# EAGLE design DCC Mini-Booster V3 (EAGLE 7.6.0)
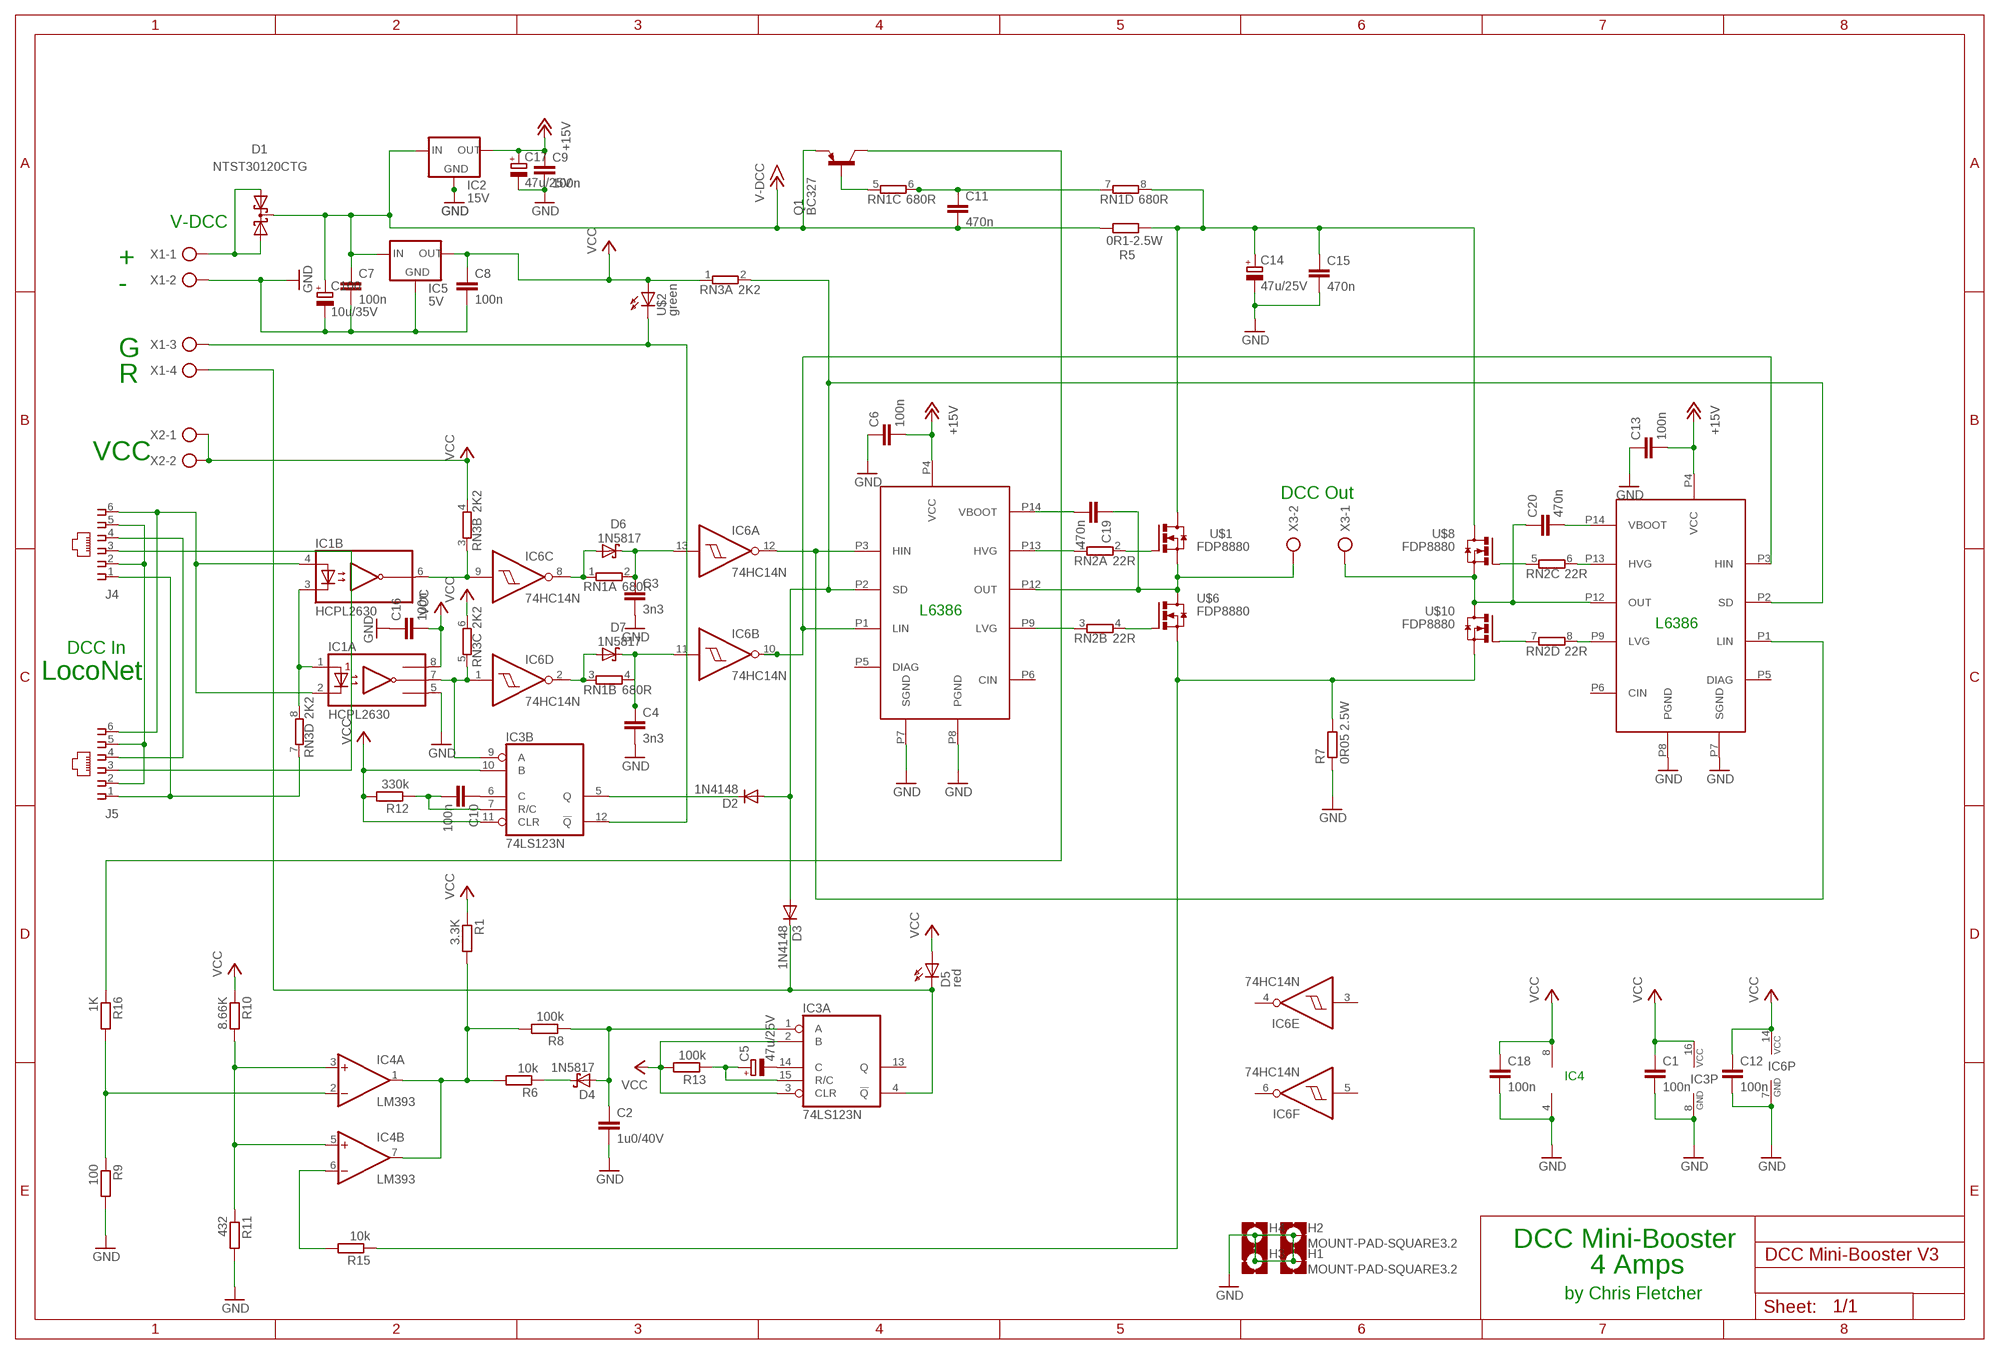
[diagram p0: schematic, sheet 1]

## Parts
C1  100n  C-EU050-025X075  [C050-025X075]
C2  1u0/40V  C5/5.5  [C5B5.5]
C3  3n3  C-EU050-025X075  [C050-025X075]
C4  3n3  C-EU050-025X075  [C050-025X075]
C5  47u/25V  CPOL-EUE2.5-6  [E2,5-6]
C6  100n  C-EU050-025X075  [C050-025X075]
C7  100n  C-EU050-025X075  [C050-025X075]
C8  100n  C-EU050-025X075  [C050-025X075]
C9  100n  C-EU050-025X075  [C050-025X075]
C10  100n  C-EU050-025X075  [C050-025X075]
C11  470n  C-EU050-025X075  [C050-025X075]
C12  100n  C-EU050-025X075  [C050-025X075]
C13  100n  C-EU050-025X075  [C050-025X075]
C14  47u/25V  CPOL-EUE2.5-6  [E2,5-6]
C15  470n  C-EU050-025X075  [C050-025X075]
C16  100n  C-EU050-025X075  [C050-025X075]
C17  47u/25V  CPOL-EUE2.5-6  [E2,5-6]
C18  100n  C-EU050-025X075  [C050-025X075]
C19  470n  C-EU050-025X075  [C050-025X075]
C20  470n  C-EU050-025X075  [C050-025X075]
C100  10u/35V  CPOL-EUE5-4  [E5-4]
D1  NTST30120CTG  DIODE_2SCHOTTKY-SOT82V  [SOT82S]
D2  1N4148  [DO35-10]
D3  1N4148  [DO35-10]
D4  1N5817  1N5817-B  [DO41-7.6]
D5  red  LED3MM  [LED3MM]
D6  1N5817  1N5817-B  [DO41-7.6]
D7  1N5817  1N5817-B  [DO41-7.6]
H1  MOUNT-PAD-SQUARE3.2  [3,2-PAD-SQUARE]
H2  MOUNT-PAD-SQUARE3.2  [3,2-PAD-SQUARE]
H3  MOUNT-PAD-SQUARE3.2  [3,2-PAD-SQUARE]
H4  MOUNT-PAD-SQUARE3.2  [3,2-PAD-SQUARE]
IC1  HCPL2630  [DIL08]
IC2  15V  78XXS  [78XXS]
IC3  74LS123N  [DIL16]
IC4  LM393  [DIL08N]
IC5  5V  78XXS  [78XXS]
IC6  74HC14N  [DIL14]
J4  520258-3  [520258-3]
J5  520258-3  [520258-3]
Q1  BC327  [TO92-EBC]
R1  3.3K  R-EU_0207/10  [0207/10]
R5  0R1-2.5W  R-EU_0613/5V  [P0613V]
R6  10k  R-EU_0207/10  [0207/10]
R7  0R05 2.5W  R-EU_0613/5V  [P0613V]
R8  100k  R-EU_0207/10  [0207/10]
R9  100  R-EU_0207/10  [0207/10]
R10  8.66K  R-EU_0207/10  [0207/10]
R11  432  R-EU_0207/10  [0207/10]
R12  330k  R-EU_0207/10  [0207/10]
R13  100k  R-EU_0207/10  [0207/10]
R15  10k  R-EU_0207/10  [0207/10]
R16  1K  R-EU_0207/10  [0207/10]
RN1  680R  E4R  [SIL8]
RN2  22R  E4R  [SIL8]
RN3  2K2  E4R  [SIL8]
U$1  FDP8880  IRFZ44Z  [TO220AV]
U$2  green  LED3MM  [LED3MM]
U$6  FDP8880  IRFZ44Z  [TO220AV]
U$7  L6386  [DIL14-1]
U$8  FDP8880  IRFZ44Z  [TO220AV]
U$9  L6386  [DIL14-1]
U$10  FDP8880  IRFZ44Z  [TO220AV]
X1  + - G R  AK500/4  [AK500/4]
X2  AK500/2  [AK500/2]
X3  AK500/2  [AK500/2]

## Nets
+12V [+15V]: C6.2 C9.1 C13.2 C17.+ IC2.OUT U$7.P4(VCC) U$9.P4(VCC) ; supply symbol labelled +15V
+15V [+VDCC]: C7.1 C11.2 C100.+ D1.C IC2.IN IC5.IN Q1.E R5.1 ; supply symbol labelled V-DCC
C10: C10.2 IC3.7(B:R/C) R12.1
GND [GND]: C1.2 C2.2 C3.2 C4.2 C6.1 C7.2 C8.2 C9.2 C12.2 C13.1 C14.- C15.2 C16.1 C17.- C18.2 C100.- H1.B3,2(MOUNT) H2.B3,2(MOUNT) H3.B3,2(MOUNT) H4.B3,2(MOUNT) IC1.5(A:GND) IC2.GND IC3.8(P:GND) IC4.4(P:V-) IC5.GND IC6.7(P:GND) R7.1 R9.2 R11.2 U$7.P7(SGND) U$7.P8(PGND) U$9.P7(SGND) U$9.P8(PGND) X1.2
N$1: IC4.1(A:OUT) IC4.7(B:OUT) R1.2 R6.2 R8.2
N$2: D4.C R6.1
N$3: C2.1 D4.A IC3.1(A:A) R8.1
N$4: C11.1 RN1.6 RN1.7
N$5: C20.2 U$9.P14(VBOOT)
N$6 [signal]: D6.A IC6.8(C:O) RN1.1
N$7: C5.- IC3.14(A:C)
N$8 [signal]: C3.1 D6.C IC6.13(A:I) RN1.2
N$9 [+VDCC]: R7.2 R15.1 U$6.E(S) U$10.E(S)
N$10 [signal]: J4.2 J4.5 J5.2 J5.5
N$11 [signal]: IC1.2(A:C1) IC1.4(B:A2) J4.6 J5.6
N$12: IC1.7(A:VO1) IC3.9(B:A) IC6.1(D:I) RN3.5
N$13 [signal]: J4.3 J5.3
N$14 [signal]: J4.1 J5.1 RN3.7
N$15: IC4.3(A:+IN) IC4.5(B:+IN) R10.2 R11.1
N$16 [signal]: J4.4 J5.4
N$17: IC4.6(B:-IN) R15.2
N$18: IC3.12(B:!Q) U$2.K(C) X1.3
N$19: Q1.C R16.1
N$20 [+VDCC]: C19.1 U$1.E(S) U$6.C(D) U$7.P12(OUT) X3.2
N$21: C4.1 D7.C IC6.11(B:I) RN1.4
N$22: D2.A D3.A RN3.2 U$7.P2(SD) U$9.P2(SD)
N$23 [signal]: IC6.12(A:O) U$7.P3(HIN) U$9.P1(LIN)
N$24: IC4.2(A:-IN) R9.1 R16.2
N$26 [+VDCC]: D1.A1 D1.A2 X1.1
N$28: IC1.1(A:A1) IC1.3(B:C2) RN3.8
N$29 [GND]: C14.+ C15.1 R5.2 RN1.8 U$1.C(D) U$8.C(D)
N$31: Q1.B RN1.5
N$32: RN2.2 U$1.B(G)
N$33: D7.A IC6.2(D:O) RN1.3
N$34 [+VDCC]: C20.1 U$8.E(S) U$9.P12(OUT) U$10.C(D) X3.1
N$35 [signal]: IC1.6(B:VO2) IC6.9(C:I) RN3.3
N$37: RN2.1 U$7.P13(HVG)
N$38: C10.1 IC3.6(B:C)
N$39: D2.C IC3.5(B:Q)
N$40: RN2.4 U$6.B(G)
N$41: RN2.3 U$7.P9(LVG)
N$42: RN2.6 U$9.P13(HVG)
N$43: C5.+ IC3.15(A:R/C) R13.1
N$44: RN2.5 U$8.B(G)
N$45: RN2.8 U$9.P9(LVG)
N$46: RN2.7 U$10.B(G)
N$47: D3.C D5.K(C) IC3.4(A:!Q) X1.4
N$48: IC6.10(B:O) U$7.P1(LIN) U$9.P3(HIN)
N$59: C19.2 U$7.P14(VBOOT)
VCC [VCC]: C1.1 C8.1 C12.1 C16.2 C18.1 D5.A IC1.8(A:VCC) IC3.2(A:B) IC3.3(A:CLR) IC3.10(B:B) IC3.11(B:CLR) IC3.16(P:VCC) IC4.8(P:V+) IC5.OUT IC6.14(P:VCC) R1.1 R10.1 R12.2 R13.2 RN3.1 RN3.4 RN3.6 U$2.A X2.1 X2.2
Unconnected: IC3.13(A:Q) IC6.3(E:I) IC6.4(E:O) IC6.5(F:I) IC6.6(F:O) U$7.P5(DIAG) U$7.P6(CIN) U$9.P5(DIAG) U$9.P6(CIN)

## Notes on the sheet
- V-DCC
- +
- -
- G
- R
- VCC
- DCC Out
- L6386
- L6386
- DCC In
- LocoNet
- IC4
- DCC Mini-Booster
- 4 Amps
- by Chris Fletcher

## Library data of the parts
C1 C3 C4 C6-C13 C15 C16 C18-C20 = rcl:C-EU: CAPACITOR, European symbol
C2 = capacitor-wima:C: CAPACITOR
C5 C14 C17 C100 = rcl:CPOL-EU: POLARIZED CAPACITOR, European symbol
D1 = diode:DIODE_2SCHOTTKY-: Dual SCHOTTKY DIODE common cathode
D2 D3 = diode:1N4148: DIODE
D4 D6 D7 = diode:1N581*: 1.0A SCHOTTKY BARRIER RECTIFIER
D5 U$2 = led:LED: LED
H1-H4 = holes:MOUNT-PAD-SQUARE: MOUNTING PAD, square
IC1 = optocoupler:HCPL2630: HEWLETT PACKARD OPTO COUPLER
IC2 IC5 = v-reg:78XXS: VOLTAGE REGULATOR
IC3 = 74xx-eu:74*123: Retriggerable monostable MULTIVIBRATOR
IC4 = linear:LM393: COMPARATOR
IC6 = 74xx-eu:74*14: Hex schmitt trigger INVERTER
J4 J5 = con-amp:520258-3: AMP connector; MF: TYCO ELECTRONICS; MPN: 5520258-3; OC_FARNELL: 1214651; OC_NEWARK: 42K7227
Q1 = transistor-pnp:BC327*: PNP Transistror
R1 R5-R13 R15 R16 = rcl:R-EU_: RESISTOR, European symbol
RN1-RN3 = resistor-sil:E4R: SIL RESISTOR; OC_FARNELL: unknown; OC_NEWARK: unknown
U$1 U$6 U$8 U$10 = transistor-power:IRFZ44Z: N-Channel MOSFET TO-220 Pack
U$7 U$9 = jfw-pwm1:L6386: High and low side MOSFET Driver
X1 = con-ptr500:AK500/4: CONNECTOR; OC_FARNELL: unknown; OC_NEWARK: unknown
X2 X3 = con-ptr500:AK500/2: CONNECTOR; OC_FARNELL: unknown; OC_NEWARK: unknown

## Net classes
1 signal: width 0.381 mm, drill 0.508 mm, clearance 0.381 mm
2 VCC: width 0.635 mm, drill 0.508 mm, clearance 0.381 mm
3 +15V: width 0.635 mm, drill 0.508 mm, clearance 0.381 mm
4 +VDCC: width 1.803 mm, drill 0.762 mm, clearance 0.381 mm
5 GND: width 0.635 mm, drill 0.508 mm, clearance 0.381 mm

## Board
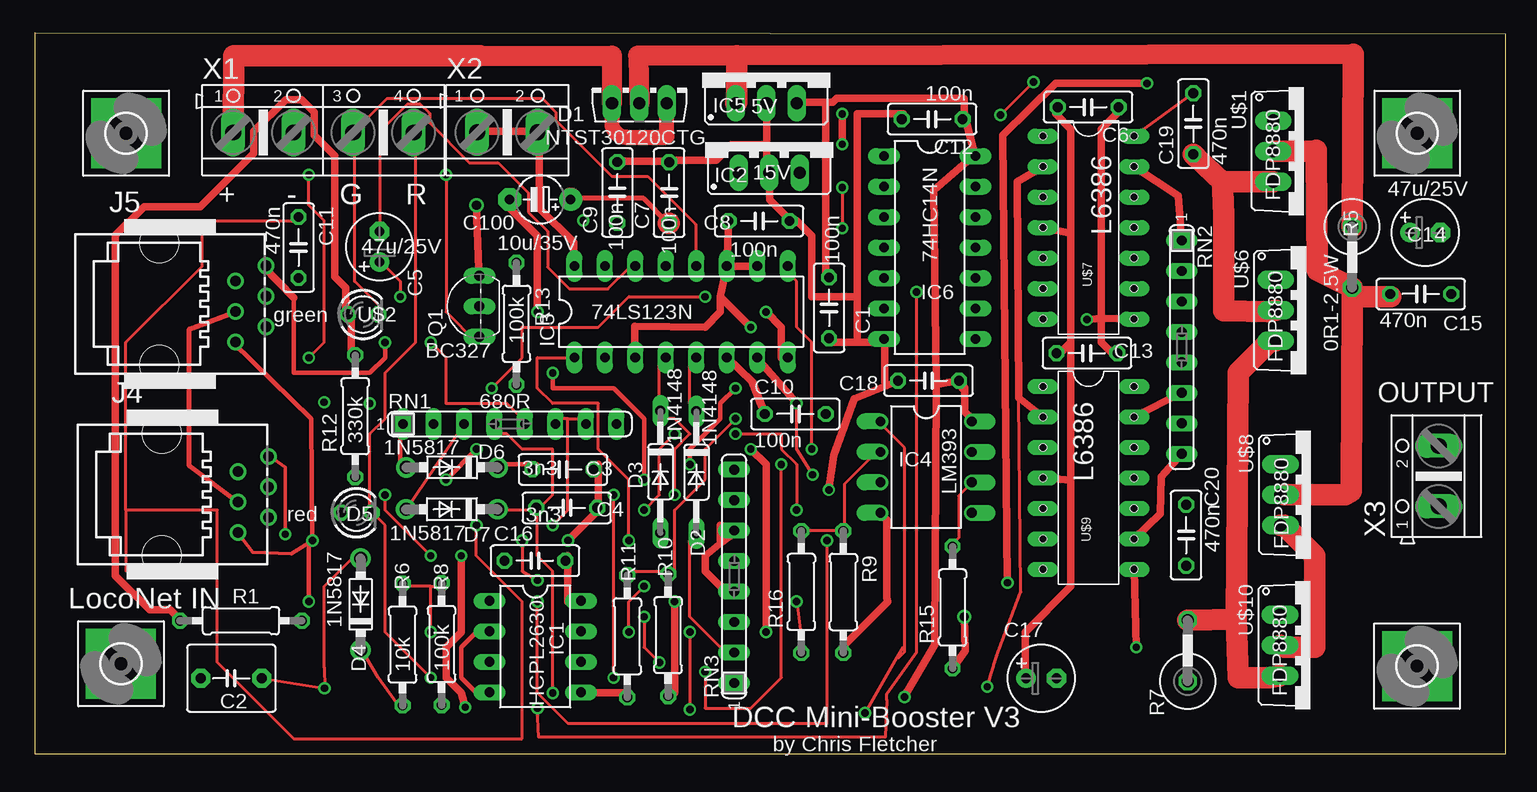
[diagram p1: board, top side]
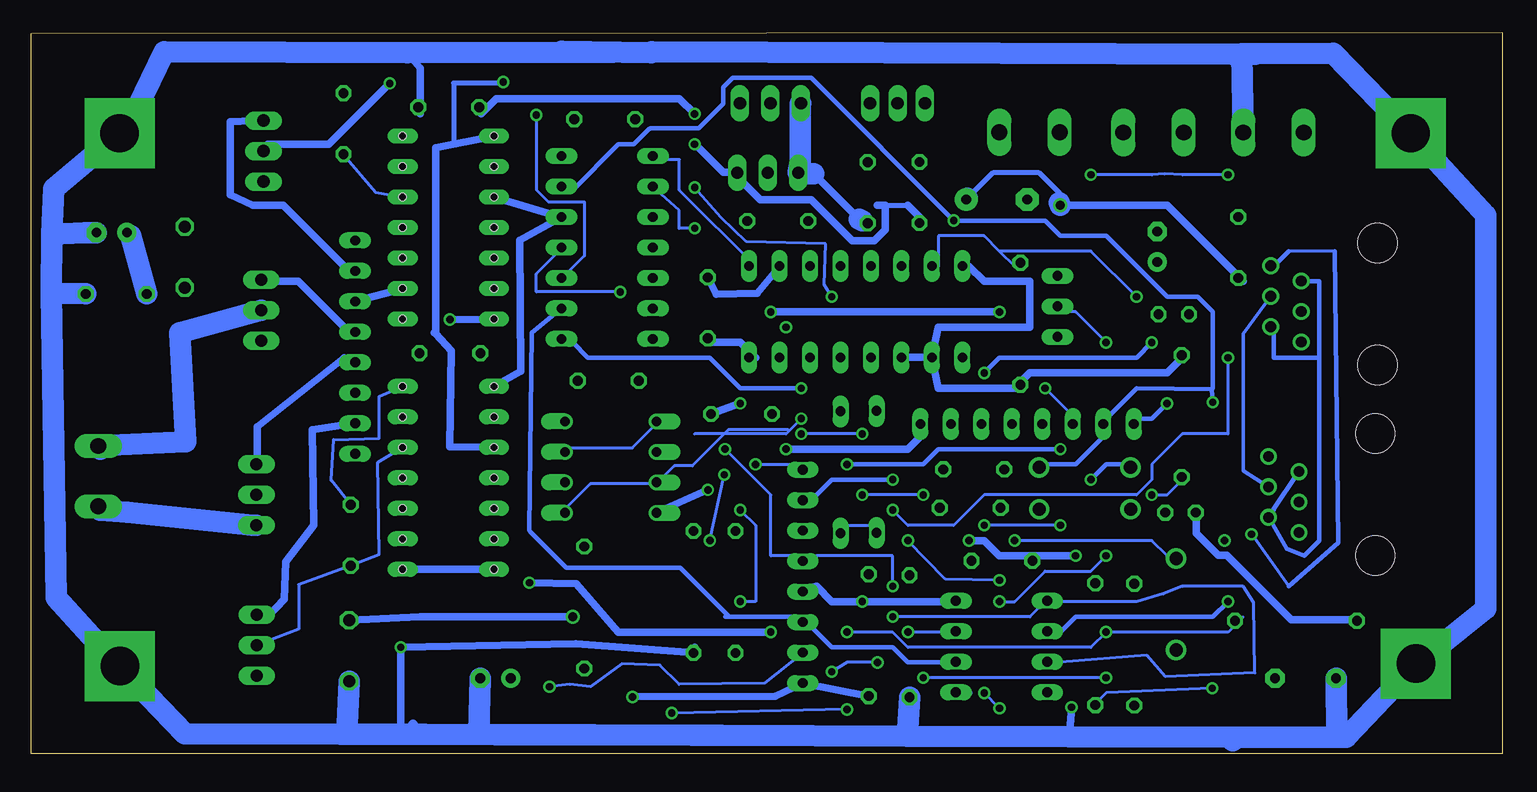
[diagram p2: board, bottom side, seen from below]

Size 122.6 x 60.1 mm. Coordinates in mm from the lower left corner, seen from the top.
Outline: 122.6,0 122.6,60 0,60.1 0,0 122.6,0
Copper layers (1*16): Top 0.035mm / dielectric 1.5mm / Bottom 0.035mm
Design rules "default": minimum track width 10mil, minimum drill 24mil, track to track 8mil, track to pad 8mil, pad to pad 8mil, via to via 8mil, smd to smd 8mil, copper to edge 40mil, drill to drill 8mil, minimum pad ring 10mil, minimum via ring 8mil, stop-mask expansion 4mil, vias tented up to drill 0mil, thermal gap 10mil

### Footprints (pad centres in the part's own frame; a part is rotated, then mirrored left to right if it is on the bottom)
C050-025X075 = drill 0.813 octagon: 1 -2.54,0; 2 2.54,0
C5B5.5 = drill 0.813 pad 1.6 octagon: 1 -2.54,0; 2 2.54,0
E2,5-6 = drill 0.813 pad 1.6: + -1.27,0 | drill 0.813 pad 1.6 octagon: - 1.27,0
E5-4 = drill 0.813 pad 1.905: + -2.54,0 | drill 0.813 pad 1.905 octagon: - 2.54,0
SOT82S = drill 1.016 long: A1 -2.286,-1.27; A2 2.286,-1.27; C 0,-1.27
DO35-10 = drill 0.813 long: A 5.08,0; C -5.08,0
DO41-7.6 = drill 1.1 pad 1.7: A 3.81,0; C -3.81,0
LED3MM = drill 0.813 octagon: A -1.27,0; K 1.27,0
3,2-PAD-SQUARE = drill 3.2 pad 5.842 square: B3,2 0,0
DIL08 = drill 0.813 long: 1 -3.81,-3.81; 2 -1.27,-3.81; 3 1.27,-3.81; 4 3.81,-3.81; 5 3.81,3.81; 6 1.27,3.81; 7 -1.27,3.81; 8 -3.81,3.81
78XXS = drill 1.016 long: GND 0,-2.54; IN -2.54,-2.54; OUT 2.54,-2.54
DIL16 = drill 0.813 long: 1 -8.89,-3.81; 2 -6.35,-3.81; 3 -3.81,-3.81; 4 -1.27,-3.81; 5 1.27,-3.81; 6 3.81,-3.81; 7 6.35,-3.81; 8 8.89,-3.81; 9 8.89,3.81; 10 6.35,3.81; 11 3.81,3.81; 12 1.27,3.81; 13 -1.27,3.81; 14 -3.81,3.81; 15 -6.35,3.81; 16 -8.89,3.81
DIL08N = drill 0.813 offset: 1 -3.81,-3.81; 2 -1.27,-3.81; 3 1.27,-3.81; 4 3.81,-3.81; 5 3.81,3.81; 6 1.27,3.81; 7 -1.27,3.81; 8 -3.81,3.81
DIL14 = drill 0.813 long: 1 -7.62,-3.81; 2 -5.08,-3.81; 3 -2.54,-3.81; 4 0,-3.81; 5 2.54,-3.81; 6 5.08,-3.81; 7 7.62,-3.81; 8 7.62,3.81; 9 5.08,3.81; 10 2.54,3.81; 11 0,3.81; 12 -2.54,3.81; 13 -5.08,3.81; 14 -7.62,3.81
520258-3 = drill 0.889: 1 -3.175,8.001; 2 -1.905,5.461; 3 -0.635,8.001; 4 0.635,5.461; 5 1.905,8.001; 6 3.175,5.461 | hole 3.251: -5.08,-0.889; 5.08,-0.889
TO92-EBC = drill 0.813 long: B 0,-1.27; C -2.54,-1.27; E 2.54,-1.27
0207/10 = drill 0.813 octagon: 1 -5.08,0; 2 5.08,0
P0613V = drill 1.016 octagon: 1 -2.54,0; 2 2.54,0
SIL8 = drill 0.813 long: 1 -8.89,0; 2 -6.35,0; 3 -3.81,0; 4 -1.27,0; 5 1.27,0; 6 3.81,0; 7 6.35,0; 8 8.89,0
TO220AV = drill 1.016 long: B -2.54,-2.54; C 0,-2.54; E 2.54,-2.54
DIL14-1 = drill 0.406 pad 1.27 long: P1 -8.89,-3.81; P2 -6.35,-3.81; P3 -3.81,-3.81; P4 -1.27,-3.81; P5 1.27,-3.81; P6 3.81,-3.81; P7 6.35,-3.81; P8 6.35,3.81; P9 3.81,3.81; P10 1.27,3.81; P11 -1.27,3.81; P12 -3.81,3.81; P13 -6.35,3.81; P14 -8.89,3.81 | hole 0.61: -8.89,-3.81; -6.35,-3.81; -3.81,-3.81; -1.27,-3.81; 1.27,-3.81; 3.81,-3.81; 6.35,-3.81; 6.35,3.81; 3.81,3.81; 1.27,3.81; -1.27,3.81; -3.81,3.81; -6.35,3.81; -8.89,3.81
AK500/4 = drill 1.321 long: 1 -7.518,0; 2 -2.489,0; 3 2.489,0; 4 7.518,0
AK500/2 = drill 1.321 long: 1 -2.515,0; 2 2.515,0

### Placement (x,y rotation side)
C1  66.21,37.17 270 top
C2  16.4,6.3 180 top
C3  44.04,23.71 0 top
C4  44.35,20.51 0 top
C5  28.75,42.26 90 top
C6  87.8,53.9 180 top
C7  52.89,46.77 90 top
C8  60.38,44.41 0 top
C9  48.57,46.79 90 top
C10  63.4,28.33 0 top
C11  22,42.2 270 top
C12  74.8,52.9 180 top
C13  87.7,33.4 180 top
C14  115.89,43.45 0 top
C15  115.51,38.33 0 top
C16  41.7,16.1 0 top
C17  83.9,6.3 0 top
C18  74.5,31.1 180 top
C19  96.57,52.52 90 top
C20  95.97,18.23 90 top
C100  42.13,46.2 180 top
D1  50.4,55.5 0 top
D2  55.15,23.47 270 top
D3  52.15,23.51 270 top
D4  27.18,12.47 90 top
D5  26.82,20.11 0 top
D6  34.79,23.88 180 top
D7  34.78,20.39 180 top
H1  7.2,7.52 0 top
H2  115.21,7.32 0 top
H3  115.22,51.72 0 top
H4  7.63,51.72 0 top
IC1  41.73,8.95 270 top
IC2  61.22,50.97 0 top
IC3  53.88,36.85 0 top
IC4  74.3,23.9 270 top
IC5  60.99,56.77 0 top
IC6  74.6,42.2 270 top
J4  11.49,21.62 270 top
J5  11.29,37.5 270 top
Q1  35.8,37.3 90 top
R1  17.2,11.1 0 top
R5  109.8,41.4 270 top
R6  30.67,9.11 90 top
R7  96.1,8.6 90 top
R8  33.92,9.15 90 top
R9  67.4,13.5 270 top
R10  52.8,9.9 90 top
R11  49.4,9.8 270 top
R12  26.72,28.15 90 top
R13  40.16,35.85 270 top
R15  76.5,12.2 90 top
R16  63.9,13.5 90 top
RN1  39.6,27.5 0 top
RN2  95.6,33.9 270 top
RN3  58.3,14.8 90 top
U$1  105.77,50.24 270 top
U$2  27.38,36.63 0 top
U$6  105.97,36.97 270 top
U$7  87.83,42.59 270 top
U$8  106.37,21.6 270 top
U$9  87.83,21.74 270 top
U$10  106.33,9.05 270 top
X1  24.07,51.79 0 top
X2  39.4,51.8 0 top
X3  117.01,23.15 90 top

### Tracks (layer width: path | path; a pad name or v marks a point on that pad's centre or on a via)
+12V  (via drill 0.61)
  Top 0.61: 86.36,22.8 U$9.P4 | 86.36,43.4 U$7.P4
  Top 0.635: 86.36,34.29 85.09,33.02 C13.2 | 86.36,34.29 86.36,43.4 86.36,52.07 85.09,53.34 C6.2 | 86.36,34.29 86.36,22.8 86.36,13.97 82.55,10.16 82.55,6.35 C17.+ | v67.31,53.34 v67.31,50.8
  Bottom 0.406: 51.44,45.72 49.53,45.72
  Bottom 0.635: 49.53,45.72 48.26,44.45 C9.1 | 52.07,45.72 51.44,45.72 51.44,43.66 52.35,42.75 54.18,42.75 57.61,46.18 61.84,46.18 63.78,48.12 IC2.OUT 63.78,48.46 64.92,48.46 67.21,50.75 v67.31,50.8 | v67.31,53.34 68.58,54.61 83.82,54.61 85.09,53.34 C6.2
+15V  (via drill 0.76)
  Top 0.406: 44.69,46.29 50.75,46.29 52.81,44.23
  Top 0.61: v36.83,45.72 37.03,40.37 Q1.E
  Top 1.676: 109.9,58.3 58.52,58.2 50.3,58.2 D1.C
  Top 1.778: 109.9,58.3 R5.1
  Top 1.803: 58.52,58.2 58.52,54.29 IC5.IN | 44.69,46.29 C100.+ | 52.81,44.23 C7.1
  Bottom 0.406: 36.92,45.95 36.92,46.75 38.63,48.46 42.41,48.46 44.58,46.29
  Bottom 0.61: C11.2 21.59,39.37 27.94,45.72 v36.83,45.72 | 53.34,44.45 C7.1 | 57.38,48.35 53.61,44.58
  Bottom 1.803: 57.38,48.35 58.64,48.35 IC2.IN 58.52,49.26 58.52,54.18 IC5.IN | 53.61,44.58 53.34,44.45 | 36.92,45.95 v36.83,45.72 | 44.58,46.29 C100.+
C10  (via drill 0.6, 0.61)
  Top 0.254: v29.21,21.59 29.21,20.32 v33.02,16.51 | v41.91,12.7 41.91,5.08 44.45,2.54 66.04,2.54 v66.04,17.78 | v64.84,23.26 63.5,25.4 v63.5,29.21 | 60.19,33.02 IC3.7
  Top 0.61: v63.5,29.21 60.19,33.02
  Bottom 0.254: R12.1 26.67,22.86 27.94,21.59 v29.21,21.59 | v33.02,16.51 34.29,15.24 38.1,15.24 40.64,12.7 v41.91,12.7 | v66.04,17.78 v64.84,23.26
  Bottom 0.61: v63.5,29.21 C10.2
GND  (via drill 0.6, 0.61)
  Top 0.61: U$7.P8 88.9,36.3 v87.7,36.2 | 35.56,5.08 v35.9,3.9 | v91.8,8.9 U$9.P8 | C18.2 70.98,30.7 68.3,29.6 66.6,24.9 v66.2,22
  Top 0.635: 68.58,34.29 66.04,34.29 C1.2 | 68.58,34.29 69.85,34.29 IC6.7 70.87,34.29 70.87,30.98 70.98,30.7 | 68.58,38.1 68.58,34.29 | 68.58,38.1 68.58,53.34 72.39,53.34 C12.2 | v41.91,36.83 41.91,43.18 39.37,45.72 C100.- | v60.96,36.83 62.23,35.56 62.23,33.02 IC3.8 | C13.1 90.17,33.02 88.9,34.29 88.9,36.3 88.9,52.07 90.17,53.34 C6.1 | v44.45,17.78 46.99,20.32 | 46.99,20.32 46.99,24.13 C3.2 | 46.99,20.32 C4.2 | R9.2 67.31,8.89 71.12,12.7 71,13 71,19.5 70.5,20 IC4.4 | R11.2 49.53,5.08 45.72,5.08 IC1.5 | 85.09,6.35 C17.- | v35.56,16.51 35.56,10.16 34.29,8.89 34.29,6.35 35.56,5.08 | 68.58,38.1 64.77,38.1 64.77,43.18 63.5,44.45 C8.2 62.75,44.69 61.27,46.18 61.27,48.12 IC2.GND 61.15,48.46 61.04,48.58 61.04,50.75 | C9.2 48.58,49.38 52.81,49.38 C7.2 53.15,49.49 56.81,49.49 58.06,50.75 61.04,50.75 | 61.04,50.75 61.04,54.18 IC5.GND
  Bottom 0.406: 70.9,58.5 69.9,58.1 | 69.7,58.1 69.9,58.1 | 69.9,58.1 70.7,58.2
  Bottom 0.61: v35.9,3.9 36.1,1.45 | v87.7,36.2 U$7.P7 | U$9.P7 U$9.P8 | R9.2 77.2,9.2 v91.8,8.9 91.8,1.64 | v66.2,22 IC4.4
  Bottom 0.635: 115.59,7.6 115.57,7.62 H2.B3,2 | 22.66,1.44 22.45,1.11 23.16,1.44 | 65.94,1.44 83.81,1.72 85.31,1.75 90.21,1.82 91.34,1.84 90.76,2.44 | 78.38,58.55 71.12,58.42 | 74.12,58.49 77.47,58.4 77.67,58.45 | 118.12,43.41 118.11,43.18 | IC3.8 62.23,33.02 63.5,34.29 66.04,34.29 C1.2 | v60.96,36.83 v41.91,36.83 | 39.37,16.51 41.91,16.51 43.18,17.78 v44.45,17.78 | 44.45,5.08 IC1.5 | C17.- 85.09,6.35 | v35.56,16.51 39.37,16.51 | 39.37,16.51 C16.1 | C6.1 90.17,53.34 90.17,57.15 91.28,58.43 | 67.31,8.89 R9.2 | H3.B3,2 115.44,50.52 115.1,51.3 | 22.5,58.31 22.5,58.5 21.7,58.35
  Bottom 0.813: 91.5,1.64 90.76,2.44
  Bottom 1.778: H1.B3,2 7.55,7.15 | 7.55,7.15 13,1.4 13.8,1.4 | 13.8,1.4 22.2,1.4 | H3.B3,2 120.7,47.1 120.86,43.3 | 120.92,38.41 120.86,43.3 | 120.92,38.41 120.5,13 115.59,7.6 114.75,6.84 109.8,1.7 96.8,1.66 96.3,1.65 | 7.55,7.15 1.4,12.1 1.4,44.9 H4.B3,2 14.1,58.4 21.7,58.35 X1.2 | 22.2,1.4 22.45,1.11 | 120.86,43.3 118.12,43.41 C14.- | 120.92,38.41 C15.2 | 49.6,1.49 49.2,1.49 36.1,1.45 22.7,1.4 22.2,1.4 | 49.6,1.49 65.1,1.55 67.5,1.55 75.7,1.58 78.7,1.59 83.9,1.61 89.8,1.63 91.5,1.64 91.8,1.64 96.3,1.65 | 70.9,58.45 78.38,58.55 74.12,58.49 91.28,58.43 111.5,58.5 114.9,51.5 115.1,51.3 | 96.3,1.65 R7.1 | R11.2 49.6,1.49 | C2.2 13.8,1.4 | C17.- 85.31,1.75 | 20.6,58.3 22.5,58.31 70.9,58.5
N$1  (via drill 0.61)
  Top 0.254: 33.02,13.97 34.29,13.97 R8.2 | 33.02,13.97 30.48,13.97 R6.2 | v33.02,10.16 33.02,13.97 | v54.61,10.16 v54.61,3.71 | v69.21,3.41 71.91,8.05 | 71.91,8.05 72.39,8.89 | 71.91,8.05 72,8 72.5,8.5 72.5,25.5 70.5,27.5 IC4.1
  Bottom 0.254: v54.61,10.16 50.8,10.16 49.53,8.89 34.29,8.89 v33.02,10.16 22.86,10.16 21.59,11.43 R1.2 | v54.61,3.71 v69.21,3.41 | IC4.1 70.5,27.5 72.5,25.5 78,25.5 IC4.7
N$2
  Top 0.254: D4.C 27.14,8.89 28.64,6.35 30.48,3.81 R6.1
N$3  (via drill 0.61)
  Top 0.254: D4.A 26.67,16.51 24.13,13.97 24.13,7.22 v24.17,5.48 C2.1 | v49.53,17.78 49.53,22.86 46.99,25.4 46.99,29.21 43.18,29.21 41.91,30.48 41.91,33.02 44.45,33.02 IC3.1 | v41.91,14.47 40.64,15.24 v40.64,17.78
  Bottom 0.254: v24.17,5.48 33.02,5.08 34.29,3.81 R8.1 | v49.53,17.78 46.42,14.57 v41.91,14.47 | v40.64,17.78 29.21,17.78 27.94,16.51 D4.A
N$4  (via drill 0.61)
  Top 0.254: 44.45,27.94 45.72,27.94 RN1.7 | 44.45,27.94 43.18,27.94 RN1.6 | 7.62,20.32 7.62,15.24 | 7.62,20.32 7.62,34.29 13.97,40.64 13.97,44.45 21.59,44.45 C11.1 | v36.83,19.05 36.83,16.51 40.64,12.7 40.64,1.27 21.59,1.27 15.24,7.62 15.24,20.32 7.62,20.32 | v43.18,19.05 44.45,20.32 44.45,27.94
  Bottom 0.254: v36.83,19.05 v43.18,19.05
N$5
  Bottom 0.254: U$9.P14 93.6,29.8 93.6,26.3 97.4,26.2 97.6,22.8 C20.2
N$6  (via drill 0.61)
  Top 0.381: v58.42,30.48 57.15,29.21 57.15,27.94 54.61,25.4 v54.61,24.13 | v34.29,22.86 v36.83,25.4 | RN1.1 30.48,26.67 30.48,24.13 D6.A
  Bottom 0.381: v27.94,29.21 29.21,27.94 30.48,27.94 RN1.1 | v58.42,30.48 63.5,30.48 66.04,33.02 76.2,33.02 77.47,34.29 IC6.8 | v54.61,24.13 48.26,24.13 46.99,25.4 v36.83,25.4 | v34.29,22.86 33.02,24.13 31.75,24.13 D6.A
N$7
  Top 0.254: IC3.14 50.06,40.58 49.61,40.58 47.78,38.75 44.58,38.75 42.75,40.58 42.75,43.55 41.15,45.15 41.15,46.75 38.63,49.26 36.23,49.26 32.92,52.58 32.92,53.38 32.12,54.18 31.09,54.18 28.8,51.89 28.8,43.55 C5.-
N$8  (via drill 0.61)
  Top 0.381: C3.1 41.91,24.13 39.37,24.13 D6.C
  Bottom 0.381: v24.13,29.31 24.2,30.38 | D6.C 38.1,24.13 35.56,24.13 33.02,26.67 RN1.2 33.02,27.94 30.48,30.48 24.2,30.38 | 24.2,30.38 24.13,30.48 24.13,36.83 25.4,38.1 27.94,38.1 33.02,43.18 36.83,43.18 38.1,44.45 v45.72,44.45 45.83,44.58 57.61,56.35 64.12,56.35 64.92,55.55 64.92,54.18 66.98,52.12 70.98,52.12 71.12,52.07 72.39,50.8 73.66,50.8 77.47,46.99 IC6.13
N$9  (via drill 0.76)
  Top 0.61: v77.47,11.43 77.57,8.59 R15.1
  Top 1.778: R7.2 100.13,11.23
  Top 1.803: U$10.E 102.87,6.35 100.33,6.35 100.13,11.23 100.33,31.75 102.87,34.29 U$6.E
  Bottom 0.61: v77.47,11.43 90.17,11.43 R7.2
N$10
  Bottom 0.381: 15.24,33.02 19.05,33.02 19.05,35.56 J5.5 | 15.24,33.02 15.24,39.37 16.51,39.37 J5.2 | 15.24,33.02 15.24,17.78 16.51,16.51 17.95,17.11 19.45,19.72 19.08,20.34
  Bottom 0.406: J4.5 19.08,20.34 J4.2
N$11  (via drill 0.61)
  Top 0.305: J4.6 18.2,16.8 21.4,16.7 v23.16,17.78
  Top 0.381: J5.6 16.51,34.29 23.06,27.94 v23.16,17.78 22.86,17.78 v22.86,12.7 | IC1.4 36.83,5.08 35.56,6.35 35.56,8.89 36.83,10.16 IC1.2
  Bottom 0.381: v22.86,12.7 24.13,11.43 35.56,11.43 36.83,10.16 IC1.2
N$12  (via drill 0.61)
  Top 0.254: v49.53,10.16 49.53,12.7 v50.8,13.97 | v64.77,25.4 64.77,34.29 63.5,35.56 63.5,39.37 62.23,40.64 IC3.9
  Bottom 0.254: IC3.9 62.23,40.64 68.58,46.99 68.58,49.53 69.85,49.53 IC6.1 | v49.53,10.16 45.72,10.16 IC1.7 | v50.8,13.97 50.8,16.51 57.15,16.51 RN3.5 58.42,16.51 60.96,16.51 60.96,21.59 v64.77,25.4
N$13
  Bottom 0.305: J4.3 21.6,23.6 21.6,35 J5.3
N$14  (via drill 0.6, 0.61)
  Top 0.305: J4.1 19.6,24.8 20.9,23.9 v20.9,18.3
  Top 0.381: v50.8,22.86 50.8,27.94 48.26,30.48 43.18,30.48 v43.18,31.75 | v29.21,34.29 29.21,33.02 27.94,31.75 21.59,31.75 21.59,38 | J5.1 19.05,40.64
  Top 0.61: 19.05,40.64 21.59,38
  Bottom 0.254: 13.97,41.91 17.78,41.91 | 17.78,13.97 v20.9,18.3
  Bottom 0.381: 17.78,13.97 13.67,17.58 13.97,41.91 | 17.78,41.91 19.05,40.64 J5.1 | v50.8,22.86 55.88,22.86 57.15,21.59 RN3.7 | v43.18,31.75 41.91,33.02 30.48,33.02 v29.21,34.29
N$15  (via drill 0.61)
  Top 0.254: 53.34,15.24 49.53,15.24 R11.1 | 53.34,15.24 53.34,20.32 55.88,22.86 55.88,25.4 v58.42,27.94 | 53.34,15.24 R10.2
  Bottom 0.254: v58.42,27.94 59.43,26.93 | 59.43,26.93 59.69,26.67 67.31,26.67 | 59.43,26.93 59.5,27 64.5,27 67.5,24 69,24 70,23 IC4.3 70.5,22.5 76,22.5 78,20.5 IC4.5
N$16
  Top 0.406: J5.4 12.9,35.4 12.9,24 J4.4
N$17
  Top 0.254: R15.2 76.5,17.5 77,18 77,21.5 78,22.5 IC4.6
N$18
  Top 0.254: U$2.K 29.21,36.83 26.67,39.37 26.67,50.8 X1.3 26.63,51.89 29.38,54.63 42.29,54.63 43.43,53.49 43.43,52.81 48.12,48.12 51.09,48.12 55.09,44.12 55.09,40.69 IC3.12
N$19  (via drill 0.61)
  Top 0.254: v34.29,48.26 34.29,36.83 36.83,34.29 Q1.C | v22.86,48.26 22.86,45.72 24.13,44.45 24.13,34.29 v22.86,33.02 | v50.8,20.32 52.07,21.59 52.07,25.4 v53.34,26.67 | v58.42,26.67 62.23,26.67 62.23,25.4 63.5,24.13 v63.5,20.32 | v63.5,12.7 64,8.69 R16.1
  Bottom 0.254: v34.29,48.26 29.21,48.26 28.14,48.33 26.67,48.26 v22.86,48.26 | v22.86,33.02 22.86,26.67 26.67,26.67 29.21,24.13 29.21,22.86 30.48,21.59 43.18,21.59 45.72,19.05 49.53,19.05 v50.8,20.32 | v53.34,26.67 v58.42,26.67 | v63.5,20.32 62.23,19.05 62.23,12.7 v63.5,12.7
N$20
  Top 1.778: 99.12,44.9 99,46.99
  Top 1.803: 99.12,44.9 99.12,36.93 102.87,36.83 U$6.C | 98.96,47.69 102.77,47.69 U$1.E | 98.96,47.69 96.82,49.73 C19.1 | 99,46.99 98.96,47.69
  Bottom 0.254: U$7.P12 93.9,46.8 C19.1
  Bottom 1.778: U$6.C 110.2,35.1 109.7,26 X3.2
  Bottom 1.803: X3.2 116.84,25.4
N$21  (via drill 0.61)
  Top 0.254: 41.91,20.32 43.18,21.59 43.18,25.4 40.64,25.4 39.37,26.67 38.1,26.67 RN1.4 | v43.18,5.08 43.18,15.24 41.91,16.51 41.91,20.32 | 41.91,20.32 39.37,20.32 D7.C | 41.91,20.32 C4.1 | v73.5,38.5 73.5,8.5 71,5 71,4.5 70.9,1.4 42,1.4 v41.91,3.81
  Bottom 0.254: v41.91,3.81 v43.18,5.08 | v73.5,38.5 80.5,38.5 80.5,40 78.5,42 IC6.11
N$22  (via drill 0.6)
  Top 0.254: RN3.2 57.15,8.89 54.61,11.43 54.61,17.78 D2.A | 82,29.7 82.2,13.5 80.2,8.2 v79.4,5.6
  Top 0.61: U$7.P2 81.9,47.7 82,29.7 U$9.P2
  Bottom 0.254: D3.A 52.07,19.05 54.61,19.05 D2.A | RN3.2 61.5,5.9 68.6,5.8 70.2,7.4 73.4,7.5 76,5.6 77.7,5.8 v79.4,5.6
N$23
  Bottom 0.61: U$7.P3 IC6.12 81.9,42.8 81.8,31.9 U$9.P1
N$24
  Top 0.254: 67.51,18.65 64,18.65 R16.2 | 67.51,18.65 67.51,21.5 | 67.51,21.5 67.51,21.59 | 67.51,18.65 R9.1 | 67.51,21.5 67.5,21.5 67.5,22.5 70,25 IC4.2
N$26
  Top 1.27: D1.A1 48.11,52.59 arc90 49.3,51.4 52.6,51.4 arc90 52.7,51.5 52.7,54.22 arc90 D1.A2
  Top 1.676: 37.1,58.2 48.11,58.2 D1.A1
  Top 1.778: X1.1 16.6,58.2 37.1,58.2
N$28  (via drill 0.61)
  Top 0.254: v62.23,24.13 62.23,6.35 59.69,3.81 55.88,3.81 v55.88,6.85 | v52.07,7.62 50.8,8.89 v50.8,11.43
  Bottom 0.254: IC1.3 36.83,7.62 29.64,8.22 28.07,6.45 20.62,6.75 20.72,12.6 21.59,13.97 26.67,13.97 28.24,13.34 30.48,12.7 36.83,12.7 IC1.1 38.1,12.7 39.37,11.43 v50.8,11.43 | v62.23,24.13 58.42,24.13 RN3.8 | v55.88,6.85 54.61,7.62 v52.07,7.62
N$29  (via drill 0.61)
  Top 0.635: 104.14,21.59 U$8.C | 106.8,50.3 106.68,50.8 | 113.03,38.1 C15.1 | 109.8,38.1 110.49,38.1 | v59.69,25.4 60.96,24.13 v60.96,10.16 | v81.08,14.27 80.68,51.57 85.09,55.88 v92.71,55.88
  Top 1.778: 106.8,50 106.9,40.3 R5.2 | 106.8,50 106.8,50.3 | U$1.C 106.8,50.24 106.8,50 | 110.49,38.1 113.03,38.1
  Top 1.803: 104.14,21.59 109.22,21.59 109.72,21.9 109.8,38.1 R5.2
  Bottom 0.635: 104.14,21.59 U$8.C 102.87,21.59 | 114.3,43.18 C14.+ | v59.69,25.4 49.53,25.4 48.26,26.67 RN1.8 | v60.96,10.16 73.66,10.16 77.17,14.17 v81.08,14.27 | v92.71,55.88 97.79,50.8 102.87,50.8 U$1.C
  Bottom 1.778: C15.1 114.3,43.18
N$31  (via drill 0.61)
  Top 0.254: v33.02,34.29 34.29,33.02 34.29,29.21 39.37,29.21 40.64,27.94 RN1.5
  Bottom 0.254: v33.02,34.29 35.56,36.83 36.83,36.83 Q1.B
N$32
  Bottom 0.254: RN2.2 96.52,40.64
  Bottom 0.61: U$1.B 104.14,52.77 106.01,52.67 106.01,46.59 104.14,45.72 101.6,45.72 96.52,40.64
N$33  (via drill 0.6, 0.61)
  Top 0.254: 35.56,26.67 RN1.3 D7.A | v55.88,38.1 49.53,38.1 46.99,35.56 40.64,35.56 40.64,33.02 v38.1,30.48 | v67.3,47.2 v67.3,43.8
  Bottom 0.254: v38.1,30.48 35.56,27.94 RN1.3 | 69.85,46.99 IC6.2 68.6,45.3 68.6,43.8 v67.3,43.8 | v55.88,38.1 56.5,39.1 56.4,42.5 63,42.7 65.1,44.7 v67.3,47.2
N$34
  Top 1.803: U$10.C 104.14,8.89 106.68,8.89 106.68,16.51 104.14,19.05 U$8.E
  Bottom 0.254: U$9.P12 93.7,24.3 93.6,16.6 C20.1 100.3,14.1 100.3,10.4 U$10.C
  Bottom 1.803: X3.1 116.84,20.32 114.57,20.15 104.14,19.05 U$8.E
N$35
  Bottom 0.381: 58.42,11.43 55.88,8.89 50.8,8.89 49.53,7.62 45.72,7.62 IC1.6 | 58.42,11.43 64.5,11.43 | 64.5,11.43 64.77,11.43 | IC6.9 78.74,36.83 80.88,35.09 81.08,18.64 81,18.5 78,15.5 68.5,15.5 64.5,11.5 64.5,11.43 | 58.42,11.43 RN3.3
N$37
  Top 0.61: U$7.P13 95.3,46.5 RN2.1
N$38
  Top 0.61: C10.1 59.8,31 IC3.6
N$39
  Top 0.254: D2.C 54.61,29.21 54.61,33.02 IC3.5
N$40
  Bottom 0.254: 102.87,39.37 U$6.B | RN2.4 96.52,35.56
  Bottom 0.61: 102.87,39.37 100.33,39.37 96.52,35.56
N$41
  Bottom 0.61: RN2.3 U$7.P9
N$42
  Top 0.61: U$9.P13 RN2.6
N$43  (via drill 0.61)
  Top 0.254: v30.48,38.1 30.48,39.37 29.21,40.64 C5.+
  Bottom 0.254: 41.91,41.91 40.64,40.64 R13.1 | 41.91,41.91 43.18,43.18 46.99,43.18 46.99,40.64 IC3.15 | v30.48,38.1 34.29,41.91 41.91,41.91
N$44
  Bottom 0.254: 103.77,24.73 U$8.B | RN2.5 96.52,33.02
  Bottom 0.61: 103.77,24.73 103.77,27.27 96.52,33.02
N$45
  Top 0.61: U$9.P9 93.8,20 93.9,23.1 RN2.8
N$46
  Bottom 0.254: U$10.B 102.87,11.43 | 95.62,27.54 RN2.7
  Bottom 0.61: 102.87,11.43 101.5,12.9 101.4,16.01 99.06,19.05 99.16,27 95.62,27.54
N$47  (via drill 0.61)
  Top 0.254: IC3.4 52.07,33.02 52.07,29.21 D3.C 52.07,27.94 53.34,27.94 54.61,26.67 53.34,25.4 v53.34,21.59 | 27.94,20.32 27.94,26.67 29.21,27.94 29.21,31.75 31.75,34.29 31.75,50.8 X1.4 | v48.26,6.35 v48.26,21.59 | v33.02,6.35 29.21,10.16 29.21,19.05 27.94,20.32 | 27.94,20.32 D5.K
  Bottom 0.254: D5.K 27.94,20.32 | v48.26,21.59 v53.34,21.59 | v33.02,6.35 v48.26,6.35
N$48  (via drill 0.61)
  Top 0.254: v83.25,56 v80.5,53.25
  Bottom 0.254: v80.5,53.25 80.5,47 79.5,46 76.5,46 76.5,41.5 78.25,39.75 IC6.10 | 83.15,55.9 v83.25,56
  Bottom 0.406: 83.15,55.9 87.4,55.9 87.4,50.8 87.23,50.8 87.23,50.84
  Bottom 0.61: U$9.P3 87.7,25.6 87.6,33.6 88.9,35 89,35.1 88.9,35.2 88.9,50.5 87.23,50.84 U$7.P1
N$59
  Top 0.254: U$7.P14 C19.2
VCC  (via drill 0.61)
  Top 0.61: 77.35,30.43 C18.1 | IC3.11 C8.1 | IC3.11 57.15,38.1 | 59.69,40.64 IC3.11
  Top 0.635: U$2.A 26.17,36.33 | IC3.10 59.69,40.64 | IC3.3 50.03,33.12 50.03,35.66 55.88,35.56 57.15,36.83 57.15,38.1 v59.69,35.56 | IC1.8 44.45,12.7 44.45,16.51 C16.2 | 57.27,17.62 55.88,16.51 55.88,15.24 57.15,13.97 RN3.4 | 57.27,17.62 58.35,18.48 | v53.34,12.7 53.34,5.08 R10.1 | 66.04,39.37 C1.1 65.95,39.89 65.95,54.29 | 78.37,49.93 74.93,46.99 75.13,30.78 | 78.37,49.93 77.47,53.34 | 78.37,49.93 IC6.14 | 77.47,53.34 77.47,54.61 77.27,54.63 66.86,54.63 66.52,54.29 65.95,54.29 | 77.47,53.34 C12.1 | v72.49,4.75 75.03,9.09 75.13,30.78 | 75.13,30.78 76.87,31.08 77.35,30.43 77.5,30.5 77.5,28.5 78,28 IC4.8 | RN3.6 57.15,19.05 57.15,17.78 57.27,17.62 | 65.95,54.29 63.55,54.29 IC5.OUT | U$2.A 26.4,36.12 26.4,33.49 26.63,33.26 R12.2 | U$2.A 25.95,36.92 25.95,38.86 25.03,39.78 25.03,49.84 23.32,51.55 23.32,53.49 22.29,54.52 20.92,54.52 18.29,51.89 18.29,50.06 13.83,45.61 9.14,45.61 6.74,43.2 6.74,14.86 9.6,12 11.32,12 12.12,11.2 R1.1 | X2.1 36.92,51.89 41.83,51.89 X2.2 42.06,51.55 42.06,45.49 44.92,42.63 44.92,40.69 IC3.16
  Bottom 0.61: IC3.10 62.1,38.4 65.5,38.3 C1.1 | v72.49,4.75 60.6,4.8 RN3.1 R10.1 | IC3.2 46.99,35.56 | IC3.3 IC3.2 | IC3.2 46.99,30.48
  Bottom 0.635: 40.64,30.48 46.99,30.48 | 46.99,35.56 39.37,35.56 39.37,39.37 43.18,39.37 44.45,40.64 IC3.16 | IC3.3 49.53,33.02 | 40.64,30.48 39.37,31.75 27.94,31.75 26.67,33.02 R12.2 | 40.64,30.48 R13.2 | RN3.4 57.15,13.97 55.88,12.7 v53.34,12.7 45.72,12.7 IC1.8 | C1.1 66.04,39.37 | R1.1 12.23,11.2 17.6,11.2 22.97,16.57 23.66,16.57 25.49,18.4 25.49,20 D5.A

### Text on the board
tPlace: OUTPUT | LocoNet IN | DCC Mini-Booster V3 | by Chris Fletcher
